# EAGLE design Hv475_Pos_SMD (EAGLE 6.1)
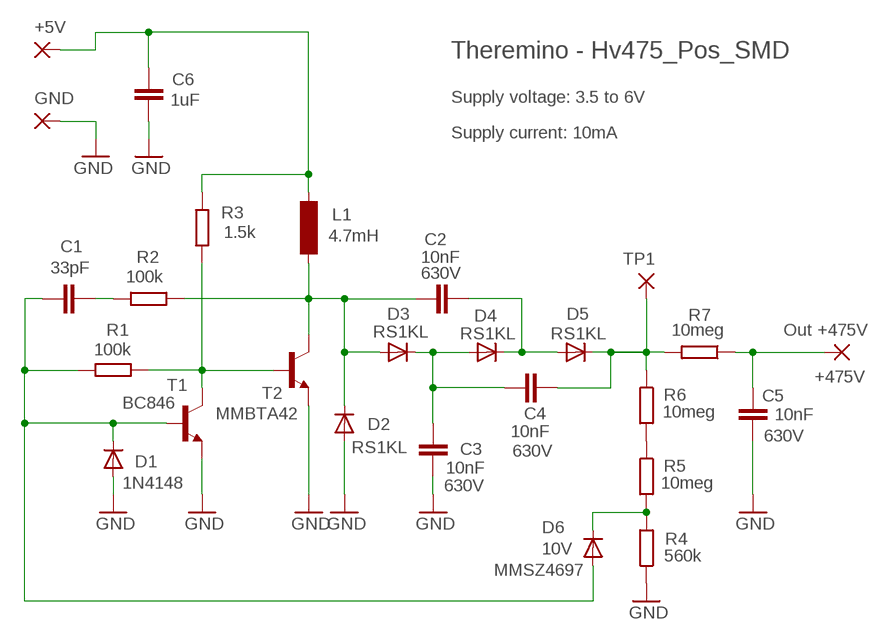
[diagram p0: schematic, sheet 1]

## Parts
+5V  WIREPADSMD5-1,8  [5-1,8]
+475V  WIREPADSMD1,90-2,54  [SMD1,90-2,54]
C1  33pF  C-EUC0805  [C0805]
C2  10nF  C-EUC1206  [C1206]
C3  10nF  C-EUC1206  [C1206]
C4  10nF  C-EUC1206  [C1206]
C5  10nF  C-EUC1206  [C1206]
C6  1uF  C-EUC0805  [C0805]
D1  1N4148  DIODE-SOD123-LARGE  [SOD123-LARGE]
D2  RS1KL  DIODE-SOD123-LARGE  [SOD123-LARGE]
D3  RS1KL  DIODE-SOD123-LARGE  [SOD123-LARGE]
D4  RS1KL  DIODE-SOD123-LARGE  [SOD123-LARGE]
D5  RS1KL  DIODE-SOD123-LARGE  [SOD123-LARGE]
D6  MMSZ4697  DIODE-SOD123-LARGE  [SOD123-LARGE]
GND  WIREPADSMD5-1,8  [5-1,8]
L1  4.7mH  INDUCTOR_4.7MH472KU  [MSD75]
R1  100k  R-EU_R0805  [R0805]
R2  100k  R-EU_R0805  [R0805]
R3  1.5k  R-EU_R1206_L  [R1206_L]
R4  560k  R-EU_R0805  [R0805]
R5  10meg  R-EU_R1206  [R1206]
R6  10meg  R-EU_R1206  [R1206]
R7  10meg  R-EU_R1206  [R1206]
T1  BC846  BC846L  [SOT23_L]
T2  MMBTA42  -NPN-BC846  [SOT23_L]
TP1  TEST  WIREPADSMD1,27-1,27  [SMD1,27-1,27]

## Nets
+5V: +5V.1(P) C6.1 L1.1 R3.2
GND: C3.1 C5.1 C6.2 D1.A D2.A GND.1(P) R4.1 T1.2(E) T2.2(E)
N$1: D6.C R4.2 R5.2
N$2: C1.2 R2.2
N$3: R5.1 R6.2
N$4: C1.1 D1.C D6.A R1.2 T1.1(B)
N$5: C4.2 D5.C R6.1 R7.2 TP1.1(P)
N$6: C2.1 D2.C D3.A L1.2 R2.1 T2.3(C)
N$11: C3.2 C4.1 D3.C D4.A
N$15: +475V.1(P) C5.2 R7.1
N$17: C2.2 D4.C D5.A
N$26: R1.1 R3.1 T1.3(C) T2.1(B)

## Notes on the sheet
- Theremino - Hv475_Pos_SMD
- Supply voltage: 3.5 to 6V
- Supply current: 10mA
- Out +475V

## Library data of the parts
+5V +475V GND TP1 = 00-LIVIO:WIREPAD: Wire PAD connect wire on PCB
C1 C6 = 00-LIVIO:C-EU: CAPACITOR, European symbol
C2-C5 = 00-LIVIO:C-EU: CAPACITOR, European symbol; VOLTAGE: 630V
D1-D5 = 00-LIVIO:DIODE-: DIODE
D6 = 00-LIVIO:DIODE-: DIODE; VZ: 10V
L1 = 00-LIVIO:INDUCTOR_4.7MH: INDUCTOR
R1-R7 = 00-LIVIO:R-EU_: RESISTOR, European symbol
T1 = 00-LIVIO:BC846
T2 = 00-LIVIO:*-NPN-: NPN Transistror

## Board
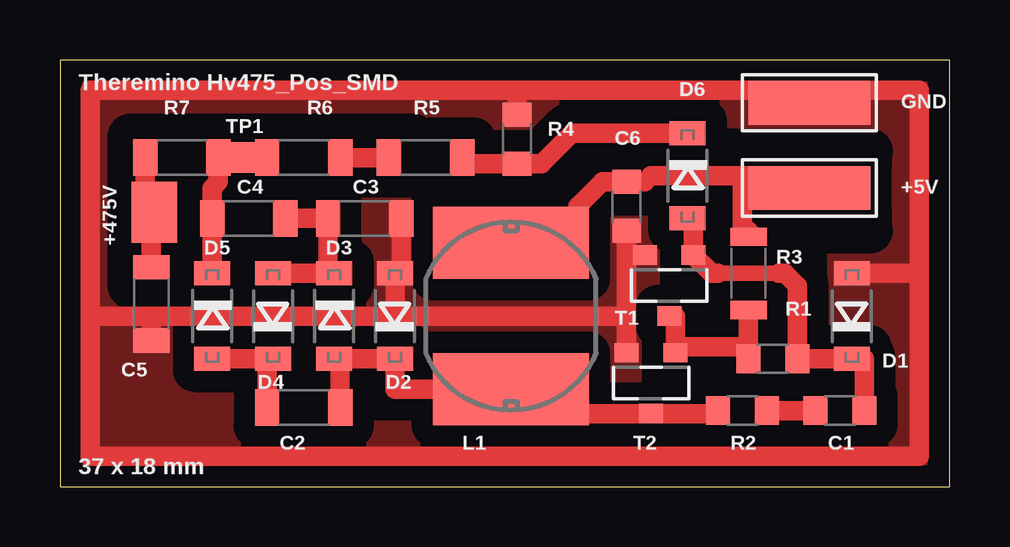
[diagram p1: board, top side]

Size 37.08 x 17.78 mm. Coordinates in mm from the lower left corner, seen from the top.
Outline: 0,0 37.08,0 37.08,17.78 0,17.78 0,0
Copper layers (1*16): Top 0.035mm / dielectric 1.5mm / Bottom 0.035mm
Design rules: minimum track width 10mil, minimum drill 27mil, track to track 27mil, track to pad 27mil, pad to pad 27mil, via to via 27mil, smd to smd 27mil, copper to edge 27mil, drill to drill 8mil, minimum pad ring 5mil, minimum via ring 8mil, stop-mask expansion 4mil, vias tented up to drill 0mil, thermal gap 41mil
tRestrict: 6 lines

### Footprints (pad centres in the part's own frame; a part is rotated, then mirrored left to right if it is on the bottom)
5-1,8 = smd 1.829 x 5.08: 1 0,0
SMD1,90-2,54 = smd 1.905 x 2.54: 1 0,0
C0805 = smd 1 x 1.2: 1 -1.016,0; 2 1.016,0
C1206 = smd 1.016 x 1.524: 1 -1.524,0; 2 1.524,0
SOD123-LARGE = smd 1 x 1.5: A 1.778,0; C -1.778,0
MSD75 = smd 3 x 6.5: 1 3.048,0; 2 -3.048,0
R0805 = smd 1 x 1.2: 1 -1.016,0; 2 1.016,0
R1206_L = smd 0.762 x 1.524: 1 -1.524,0; 2 1.524,0
R1206 = smd 1.016 x 1.524: 1 -1.524,0; 2 1.524,0
SOT23_L = smd 1 x 0.8: 1 -1.016,-1.27; 2 1.016,-1.27; 3 0,1.27
SMD1,27-1,27 = smd 1.27 x 1.27: 1 0,0

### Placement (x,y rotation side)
+5V  31.24,12.45 90 top
+475V  3.94,11.43 0 top
C1  32.51,3.17 180 top
C2  10.16,3.3 180 top
C3  12.7,11.18 180 top
C4  7.87,11.18 180 top
C5  3.81,7.62 90 top
C6  23.62,11.68 270 top
D1  33.02,7.11 90 top
D2  13.97,7.11 90 top
D3  11.43,7.11 270 top
D4  8.89,7.11 90 top
D5  6.35,7.11 270 top
D6  26.16,12.95 270 top
GND  31.24,16 90 top
L1  18.8,7.11 90 top
R1  29.72,5.33 0 top
R2  28.45,3.17 0 top
R3  28.7,8.89 90 top
R4  19.05,14.48 270 top
R5  15.24,13.72 0 top
R6  10.16,13.72 0 top
R7  5.08,13.72 0 top
T1  25.4,8.38 180 top
T2  24.64,4.32 180 top
TP1  7.62,13.72 180 top

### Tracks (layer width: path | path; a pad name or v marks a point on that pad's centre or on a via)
+5V
  Top 0.7: R3.2 28.7,10.67
  Top 0.813: L1.1 18.8,10.92 21.59,10.92 21.59,11.68 22.61,12.7 C6.1 24.38,12.7 24.64,12.95 28.45,12.95 | +5V.1 31.24,12.95 28.45,12.95 | 28.7,10.67 28.45,10.67 28.45,12.95
GND
  Top 0.813: T2.2 23.62,7.11 | 23.62,7.11 13.97,7.11 | 13.97,7.11 3.81,7.11 | 3.81,7.11 1.27,7.11 | 13.97,7.11 D2.A 14.22,8.89 C3.1 | 35.81,8.89 35.81,1.27 1.27,1.27 1.27,7.11 | 35.81,8.89 35.81,16.51 19.05,16.51 | R4.1 19.05,16.51 | 19.05,16.51 1.27,16.51 1.27,7.11 | C5.1 3.81,7.11 | T1.2 23.62,9.65 | 23.62,9.65 23.62,7.11 | D1.A 35.81,8.89 | C6.2 23.62,9.65
  pour Top (isolate 0.9, rank 6, no thermals): -1,-1 39.28,-1 39.28,18.52 -1,18.52
N$1
  Top 0.813: R5.2 16.76,13.46 R4.2 20.07,13.46 21.34,14.73 25.65,14.73 D6.C
N$2
  Top 0.813: R2.2 C1.2
N$3
  Top 0.813: R5.1 R6.2
N$4
  Top 0.65: 27.43,8.89 29.97,8.89
  Top 0.813: C1.1 33.53,5.33 D1.C | 27.43,8.89 27.18,8.89 T1.1 26.42,11.18 D6.A | 29.97,8.89 30.23,8.89 30.73,8.38 R1.2 D1.C | 33.27,5.33 D1.C
N$5
  Top 0.813: D5.C C4.2 6.35,12.45 6.6,12.7 R7.2 TP1.1 R6.1
N$6
  Top 0.813: C2.1 11.68,5.33 D3.A D2.C 13.97,4.06 L1.2 18.8,3.05 T2.3 27.43,3.05 R2.1
N$11
  Top 0.813: D4.A D3.C 11.18,8.89 C3.2 C4.1
N$15
  Top 0.813: C5.2 3.81,11.43 +475V.1 3.56,11.43 R7.1 3.56,13.97
N$17
  Top 0.813: D5.A D4.C 8.64,5.33 C2.2
N$26
  Top 0.7: 28.7,6.99 R3.1
  Top 0.813: T2.1 25.65,5.84 | 25.65,5.84 28.7,5.84 | 28.7,5.84 28.7,6.6 28.7,6.73 28.7,6.99 | R1.1 28.7,5.84 | T1.3 25.65,7.11 25.65,5.84

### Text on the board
tNames: Theremino Hv475_Pos_SMD | 37 x 18 mm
